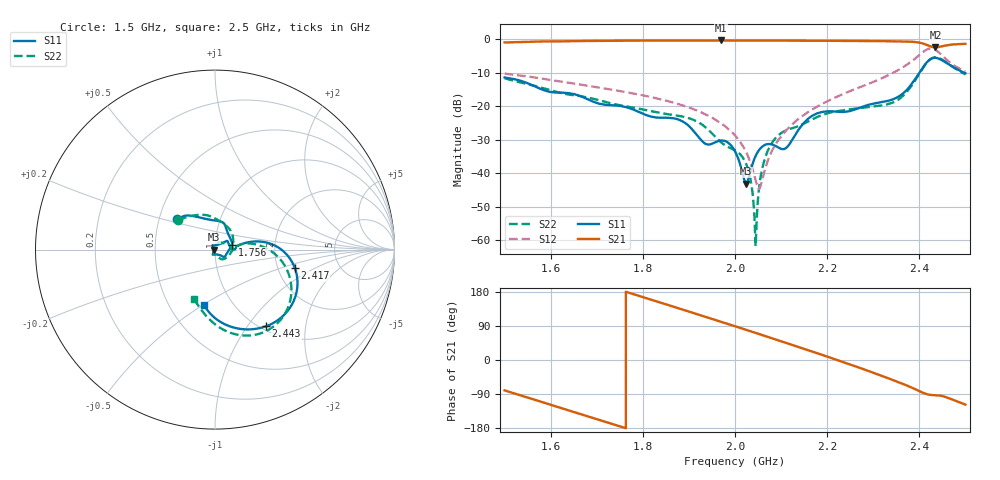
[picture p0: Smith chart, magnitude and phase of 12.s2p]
#  HZ  S  MA  R  50.00
! Rohde & Schwarz Vector Network Analyzer
! Rohde-Schwarz,ZNL6-2Port,1323001206101378,1.50.1.34-21.10.1.104
! Created: UTC 2/14/2025, 2:24:42 AM
! freq[Hz]  mag:S11  ang:S11  mag:S21  ang:S21  mag:S12  ang:S12  mag:S22  ang:S22
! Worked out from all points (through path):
!   10001 points, 1.5 GHz to 2.5 GHz, reference 50 ohm
!   highest |S21| = -0.34 dB at 1.97 GHz (marker M1); lowest = -2.4 dB at 2.435 GHz (marker M2)
!   lowest |S11| = -43.1 dB at 2.024 GHz (marker M3), VSWR 1.01, Z = 49.3 - j0.0247 ohm
!   |S11| at or under -10 dB: start of sweep to 2.4 GHz; 2.498198 GHz to end of sweep
!   |S22| runs from -61.7 to -5.4 dB; largest |S21 - S12| = 1.2
!   S11 on the Smith chart (normalised r, x): 1.5 GHz: 0.62, +0.23; 1.756 GHz: 1.21, +0.07; 2.417 GHz: 2.48, -0.65; 2.443 GHz: 1.06, -1.23; 2.5 GHz: 0.74, -0.50
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1.5e9  0.2697 140.8  0.8983 -80.1  0.3091 -109.3  0.2623 141.4
1.6667e9  0.1403 64.9  0.9432 -143.5  0.2101 -167.9  0.1411 55.8
1.7562e9  0.1 16.1  0.9531 -177.4  0.1664 160.9  0.1023 11.1
1.8334e9  0.06785 -25.6  0.958 153.3  0.13 132.5  0.08093 -29.1
1.9141e9  0.0399 -49.8  0.9609 122.4  0.08842 101.0  0.06111 -58.3
1.9704e9  0.03088 -113.2  0.9619 100.7  0.05557 78.4  0.02889 -87.0
2e9  0.02126 -116.3  0.9617 89.1  0.03679 67.8  0.02208 -111.5
2.0244e9  0.007021 -178.0  0.9611 79.6  0.02061 63.3  0.01371 -115.3
2.0342e9  0.01122 136.2  0.961 75.7  0.01414 66.4  0.007794 -112.0
2.045e9  0.0183 123.8  0.9606 71.4  0.007792 85.5  0.0008394 -16.7
2.0583e9  0.02482 121.6  0.9597 66.1  0.007575 157.6  0.01112 61.5
2.0773e9  0.02729 120.9  0.9579 58.6  0.01969 -178.8  0.02641 67.3
2.1102e9  0.02374 83.9  0.9566 45.5  0.04313 174.7  0.04357 64.5
2.1667e9  0.07166 38.0  0.9502 22.7  0.08922 148.9  0.06361 33.1
2.2499e9  0.08538 13.0  0.9444 -12.0  0.169 99.6  0.09036 7.9
2.3334e9  0.1215 7.2  0.9362 -48.5  0.2931 35.3  0.1084 3.7
2.3899e9  0.2487 10.5  0.9133 -76.3  0.5095 -34.6  0.2379 6.5
2.4167e9  0.4566 -13.0  0.8217 -90.3  0.7071 -93.6  0.452 -21.8
2.4351e9  0.5295 -44.1  0.7597 -92.8  0.697 -147.9  0.5387 -52.9
2.4426e9  0.5133 -56.3  0.7688 -93.5  0.6365 -168.7  0.5254 -64.4
2.4655e9  0.4175 -83.0  0.8269 -101.4  0.4568 140.5  0.4197 -89.3
2.5e9  0.3122 -101.5  0.8558 -117.7  0.3338 83.6  0.2997 -112.8
